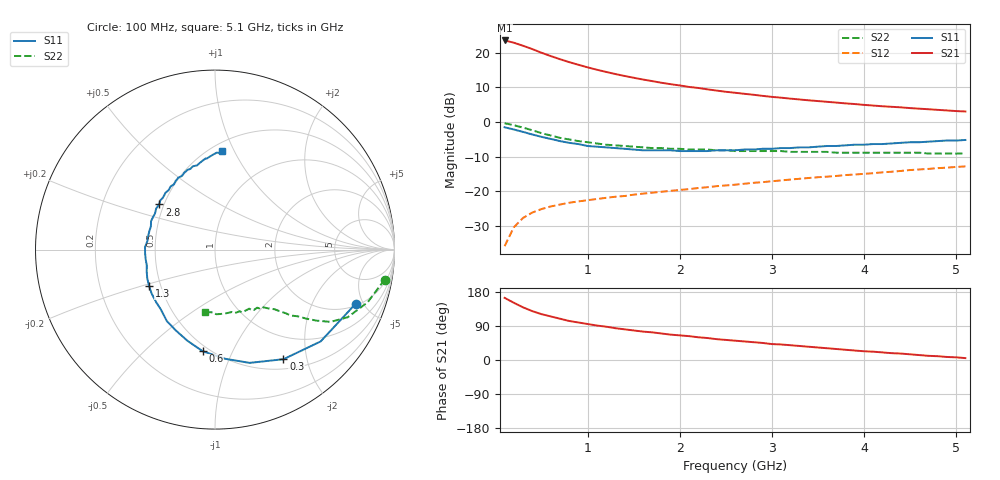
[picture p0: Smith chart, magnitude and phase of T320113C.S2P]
!AT-32011
!S PARAMETERS at Vce=2.7 V  Ic=5mA.  LAST UPDATED 01-05-95
# ghz s ma r 50
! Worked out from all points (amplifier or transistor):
!   51 points, 100 MHz to 5.1 GHz, reference 50 ohm
!   highest |S21| = 23.6 dB at 100 MHz (marker M1)
!   |S21| within 3 dB of that: start of sweep to 448 MHz
!   unconditionally stable (mu >= 1): 1.85 GHz to 5.03 GHz
!   at 900 MHz: K = 0.65, MSG = 19.8 dB, |S12| = -23.0 dB
!   at 2.6 GHz: K = 1.12, MAG = 11.2 dB, |S12| = -18.1 dB
!   at 5.1 GHz: K = 0.99, MSG = 7.9 dB, |S12| = -12.8 dB
!   S11 on the Smith chart (normalised r, x): 100 MHz: 2.15, -4.39; 300 MHz: 0.64, -1.62; 600 MHz: 0.46, -0.77; 1.3 GHz: 0.43, -0.21; 2.8 GHz: 0.47, +0.28; 5.1 GHz: 0.57, +0.90
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0.1  0.84 -21.0  15.13 164.0  0.016 79.0  0.96 -10.0
0.2  0.78 -41.0  14.04 151.0  0.03 69.0  0.9 -19.0
0.3  0.72 -58.0  12.68 139.0  0.041 62.0  0.83 -27.0
0.4  0.66 -73.0  11.36 129.0  0.049 56.0  0.76 -32.0
0.5  0.61 -85.0  10.05 121.0  0.055 52.0  0.69 -35.0
0.6  0.57 -97.0  9 115.0  0.06 50.0  0.64 -37.0
0.7  0.53 -107.0  8.11 109.0  0.064 48.0  0.59 -39.0
0.8  0.5 -116.0  7.36 103.0  0.068 47.0  0.56 -41.0
0.9  0.48 -124.0  6.73 99.0  0.071 46.0  0.53 -42.0
1  0.45 -132.0  6.18 95.0  0.074 45.0  0.51 -43.0
1.1  0.44 -138.0  5.71 91.0  0.077 45.0  0.49 -44.0
1.3  0.42 -151.0  4.95 84.0  0.083 45.0  0.46 -46.0
1.6  0.39 -167.0  4.12 75.0  0.092 45.0  0.43 -49.0
1.8  0.39 -177.0  3.7 70.0  0.098 45.0  0.42 -51.0
2.2  0.38 164.0  3.11 60.0  0.111 45.0  0.4 -56.0
2.4  0.39 156.0  2.85 55.0  0.118 45.0  0.39 -58.0
2.6  0.39 149.0  2.65 51.0  0.124 45.0  0.38 -60.0
2.8  0.4 141.0  2.48 47.0  0.132 45.0  0.38 -63.0
3  0.41 135.0  2.31 42.0  0.139 44.0  0.38 -65.0
3.5  0.44 120.0  2.01 33.0  0.159 42.0  0.37 -72.0
4.3  0.49 100.0  1.66 18.0  0.191 39.0  0.36 -83.0
5.1  0.55 86.0  1.42 5.0  0.228 33.0  0.35 -99.0
